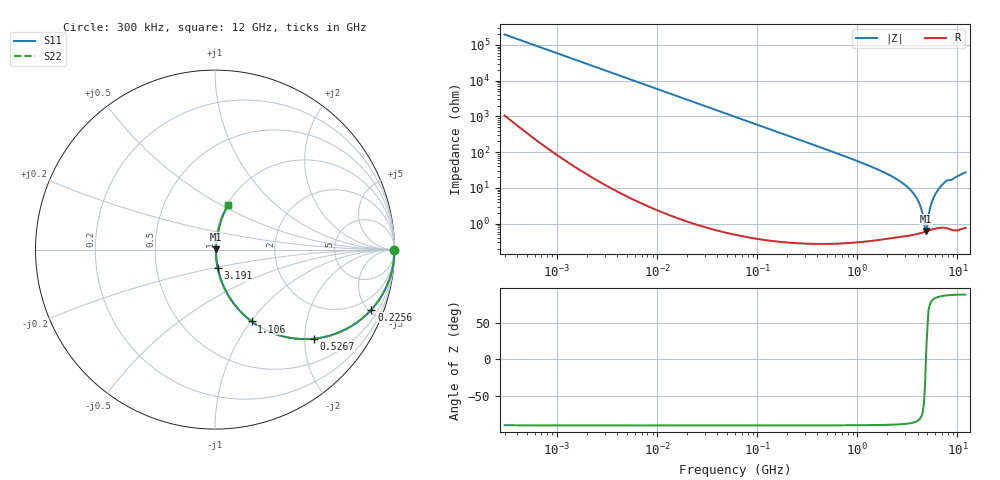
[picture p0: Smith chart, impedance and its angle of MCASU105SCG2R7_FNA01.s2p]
! MCASU105SCG2R7_FNA01  S-PARAMETER MODEL  ( Standard Model )
! Model Generated by TAIYO YUDEN Corporation (http://www.ty-top.com)
! Version 1.0
! TAIYO YUDEN Control No. 230609
! Copyright(c) 2023 TAIYO YUDEN CO.,LTD. All Rights Reserved.
! Product Description (link to TY-COMPAS)
! https://ds.yuden.co.jp/TYCOMPAS/or/detail?pn=MCASU105SCG2R7CFNA01&u=M
! Products Name : Multilayer Ceramic Capacitors
! Characteristics :
!  Capacitance : 2.7 [pF] , Rated Voltage : 50 [V] , TCC : CG / C0G
!  Case Size : 1.0 x 0.5 / 0.039 x 0.02 [mm/inch] , Thickness : 0.5 / 0.02 [mm/inch]
!  (Conditions: Temperature = 25 [degC] , DC Bias Voltage = 0 [V])
! External Node Assignments :
!  1  o---| |---o  2
! GND o---------o GND
! Frequency Range : 0.3MHz  -  12000MHz  [ 401 STEP ]
# MHZ S RI R 50
! Freq[MHz].  S11 Real  S11 Imag  S21 Real  S21 Imag  S12 Real  S12 Imag  S22 Real  S22 Imag
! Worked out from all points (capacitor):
!   401 points, 300 kHz to 12 GHz, reference 50 ohm
!   read as one part in series: C = 2.7 pF near 316.3 kHz
!   lowest |Z| = 622 mohm at 4.875 GHz (marker M1)
!   series resonance near 4.844 GHz, so ESL is about 400 pH
!   S11 on the Smith chart (normalised r, x): 300 kHz: open; 225.6 MHz: 1.01, -5.21; 526.7 MHz: 1.01, -2.21; 1.106 GHz: 1.01, -1.01; 3.191 GHz: 1.01, -0.21; 12 GHz: 1.02, +0.54
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0.3  1 -0.000509  2.99e-06 0.000509  2.99e-06 0.000509  1 -0.000509
1.769972  1 -0.003  1.16e-05 0.003  1.16e-05 0.003  1 -0.003
10.44266  0.9997 -0.0177  0.000321 0.0177  0.000321 0.0177  0.9997 -0.0177
60  0.9897 -0.1007  0.0103 0.1007  0.0103 0.1007  0.9897 -0.1007
225.6362  0.8714 -0.3342  0.1286 0.3342  0.1286 0.3342  0.8714 -0.3342
353.9943  0.7325 -0.4418  0.2675 0.4418  0.2675 0.4418  0.7325 -0.4418
526.7124  0.55 -0.4963  0.45 0.4963  0.45 0.4963  0.55 -0.4963
1105.905  0.2047 -0.4004  0.7953 0.4004  0.7953 0.4004  0.2047 -0.4004
2088.533  0.0533 -0.2163  0.9467 0.2163  0.9467 0.2163  0.0533 -0.2163
3190.978  0.0151 -0.1019  0.9849 0.1019  0.9849 0.1019  0.0151 -0.1019
3642.919  0.00958 -0.0686  0.9904 0.0686  0.9904 0.0686  0.00958 -0.0686
4050.141  0.00699 -0.0425  0.993 0.0425  0.993 0.0425  0.00699 -0.0425
4270.516  0.00626 -0.0296  0.9937 0.0296  0.9937 0.0296  0.00626 -0.0296
4623.766  0.00587 -0.0103  0.9941 0.0103  0.9941 0.0103  0.00587 -0.0103
4747.894  0.00592 -0.00389  0.9941 0.00389  0.9941 0.00389  0.00592 -0.00389
4875.354  0.00605 0.00127  0.9939 -0.00127  0.9939 -0.00127  0.00605 0.00127
5006.236  0.00623 0.00562  0.9938 -0.00562  0.9938 -0.00562  0.00623 0.00562
5565.855  0.00842 0.0396  0.9916 -0.0396  0.9916 -0.0396  0.00842 0.0396
6026.253  0.0116 0.0658  0.9884 -0.0658  0.9884 -0.0658  0.0116 0.0658
6524.734  0.0162 0.0925  0.9838 -0.0925  0.9838 -0.0925  0.0162 0.0925
7648.807  0.0298 0.1473  0.9702 -0.1473  0.9702 -0.1473  0.0298 0.1473
12000  0.0749 0.2496  0.9251 -0.2496  0.9251 -0.2496  0.0749 0.2496
